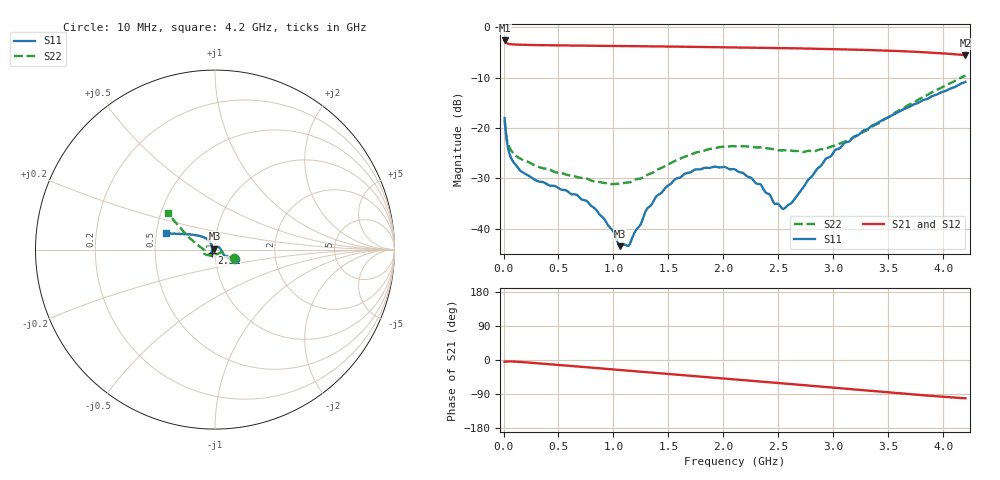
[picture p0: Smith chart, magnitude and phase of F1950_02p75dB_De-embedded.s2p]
! Integrated Device Technology
! Corporate Headquarters
! 6024 Silver Creek Valley Road
! San Jose, CA 95138  USA
! Phone:  1-408-284-8200
! Toll Free:  1-800-223-1366
! Webpage:  http://www.idt.com/
! Timing and RF Division
! 515 Groton Road, Suite 102
! Westford, MA 01886-6024
! Device:  F1950
! Description: 7-bit 0.25 dB Digital Step Attenuator
! Frequency:  150.0 -  4000.00 MHz
! Package:  4x4 mm Thin QFN Plastic Package: 24 pin
! Ports:  2 RF, 12 DC
!  Pin  1  = D0
!  Pin  2  = VDD
!  Pin  3  = Vmode
!  Pin  4  = GND
!  Pin  5  = RF1  =  Port 1
!  Pin  6  = GND
!  Pin  7  = GND
!  Pin  8  = GND
!  Pin  9  = GND
!  Pin 10  = GND
!  Pin 11  = GND
!  Pin 12  = GND
!  Pin 13  = GND
!  Pin 14  = RF2  =  Port 2
!  Pin 15  = GND
!  Pin 16  = LE
!  Pin 17  = CLK
!  Pin 18  = DATE
!  Pin 19  = D6
!  Pin 20  = D5
!  Pin 21  = D4
!  Pin 22  = D3
!  Pin 23  = D2
!  Pin 24  = D1
! State:  11
! Atten State:  2.75 dB
! Voltage:  +5.00 Volts
! Current:  Not Measured mA
! Data:  The device was measured on a the F195X evaluation board which has
!  individual transmission lines to the RF pins.  Data was collected
!  using a calibrated network analyzer.  The evaluation board was
!  de-embedded using a TRL calibration technique.
!  The reference plane is the edge of the package pin.
! Misc:  Board 2019
!  Action Tracker AT0250
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# GHz S dB R 50
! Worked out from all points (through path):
!   420 points, 10 MHz to 4.2 GHz, reference 50 ohm
!   highest |S21| = -2.62 dB at 10 MHz (marker M1); lowest = -5.5 dB at 4.2 GHz (marker M2)
!   group delay of S21, straight-line fit = 66.6 ps
!   lowest |S11| = -43.5 dB at 1.06 GHz (marker M3), VSWR 1.01, Z = 49.7 + j0.586 ohm
!   |S11| at or under -10 dB: start of sweep to end of sweep
!   |S22| runs from -31.2 to -9.6 dB; largest |S21 - S12| = 0.00082
!   S11 on the Smith chart (normalised r, x): 10 MHz: 1.25, -0.13; 2.31 GHz: 0.96, -0.04; 4.2 GHz: 0.56, +0.11
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0.01  -18.04 -25.0  -2.62 -4.5  -2.62 -4.5  -18.58 -23.1
0.06  -25.53 -28.0  -3.35 -3.7  -3.35 -3.7  -24.11 -24.2
0.15  -28.43 -13.6  -3.47 -5.1  -3.47 -5.1  -26.06 -19.3
0.71  -34.20 52.4  -3.65 -18.0  -3.65 -18.0  -29.93 -35.0
0.91  -37.92 76.3  -3.69 -22.8  -3.69 -22.8  -30.91 -53.9
1.06  -43.48 118.3  -3.73 -26.3  -3.73 -26.3  -31.08 -76.7
1.14  -43.36 164.4  -3.74 -28.2  -3.74 -28.2  -30.81 -89.0
1.3  -36.21 -150.4  -3.78 -32.0  -3.78 -32.0  -29.43 -112.5
1.41  -33.24 -140.2  -3.81 -34.7  -3.81 -34.7  -28.18 -125.2
1.56  -30.20 -133.8  -3.85 -38.2  -3.85 -38.3  -26.52 -138.2
1.74  -28.28 -128.7  -3.90 -42.6  -3.89 -42.6  -24.94 -149.5
1.92  -27.69 -126.2  -3.95 -46.9  -3.94 -46.9  -24.05 -157.7
2.11  -28.31 -126.1  -4.01 -51.4  -4.01 -51.5  -23.65 -163.3
2.31  -31.11 -134.3  -4.07 -56.2  -4.07 -56.2  -23.87 -167.5
2.46  -34.93 -154.3  -4.12 -59.8  -4.12 -59.8  -24.25 -169.9
2.55  -36.07 179.5  -4.15 -62.0  -4.15 -62.0  -24.45 -172.7
2.63  -34.61 153.2  -4.18 -63.9  -4.17 -63.9  -24.55 -173.6
2.81  -29.47 126.0  -4.25 -68.3  -4.25 -68.4  -24.66 -177.8
2.93  -26.14 123.7  -4.30 -71.3  -4.30 -71.3  -24.11 179.5
3.1  -22.99 126.3  -4.39 -75.6  -4.38 -75.6  -22.73 174.3
3.51  -17.73 141.9  -4.66 -85.7  -4.65 -85.7  -17.77 159.1
4.2  -10.85 161.2  -5.54 -101.0  -5.53 -101.1  -9.61 142.2
